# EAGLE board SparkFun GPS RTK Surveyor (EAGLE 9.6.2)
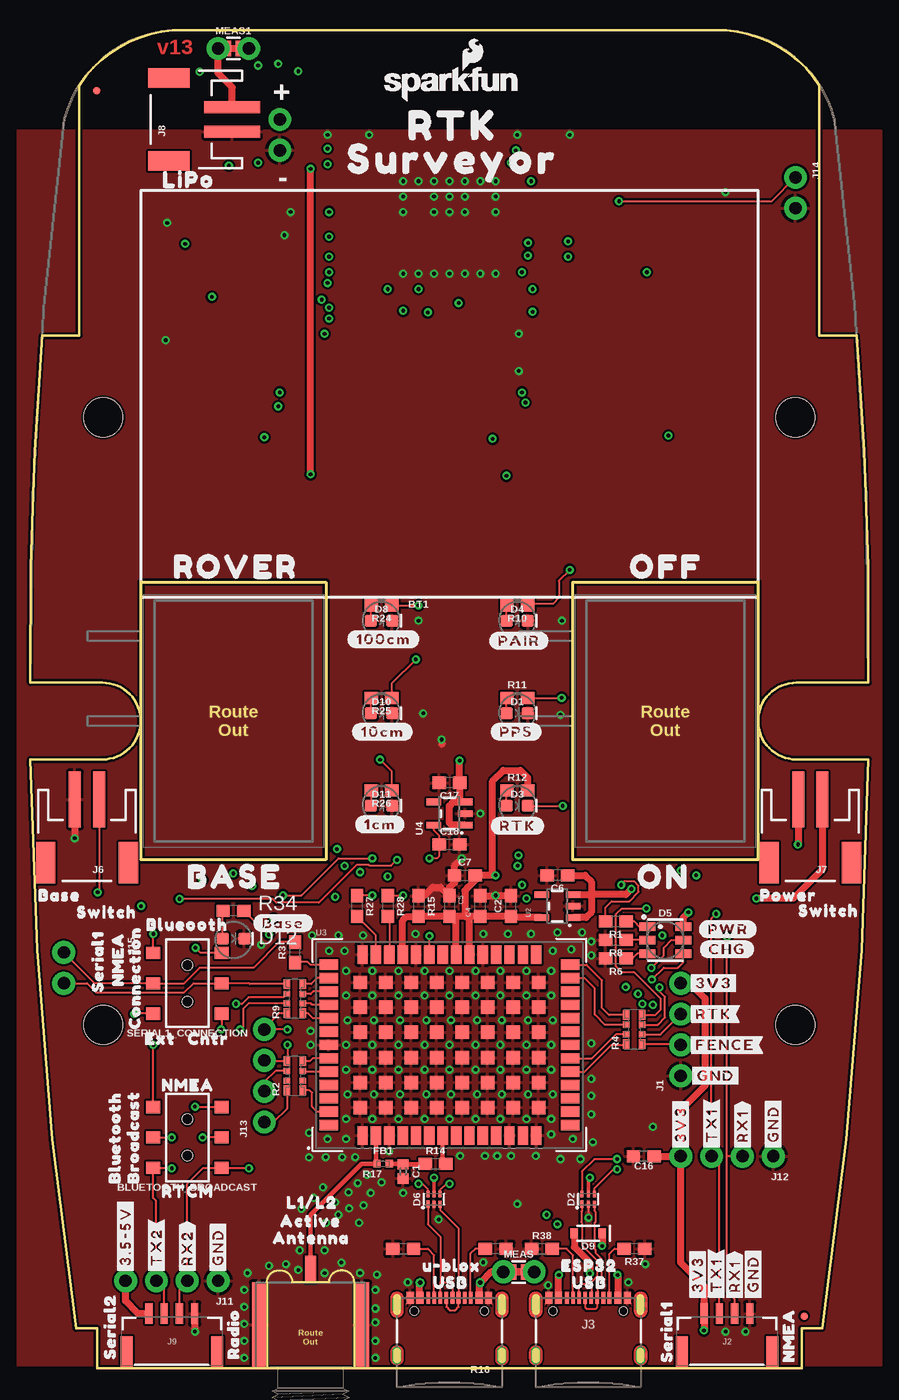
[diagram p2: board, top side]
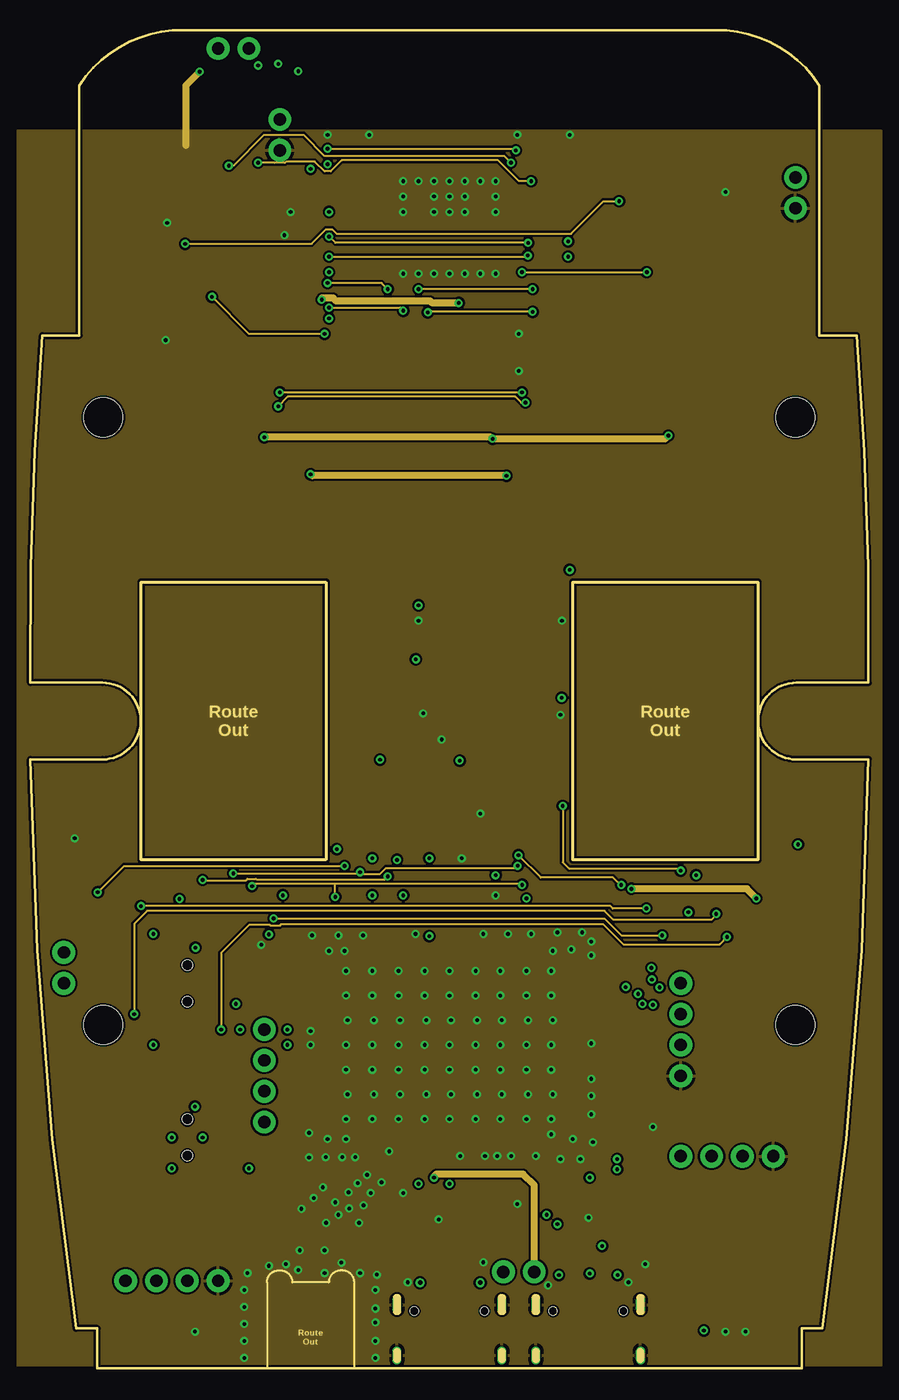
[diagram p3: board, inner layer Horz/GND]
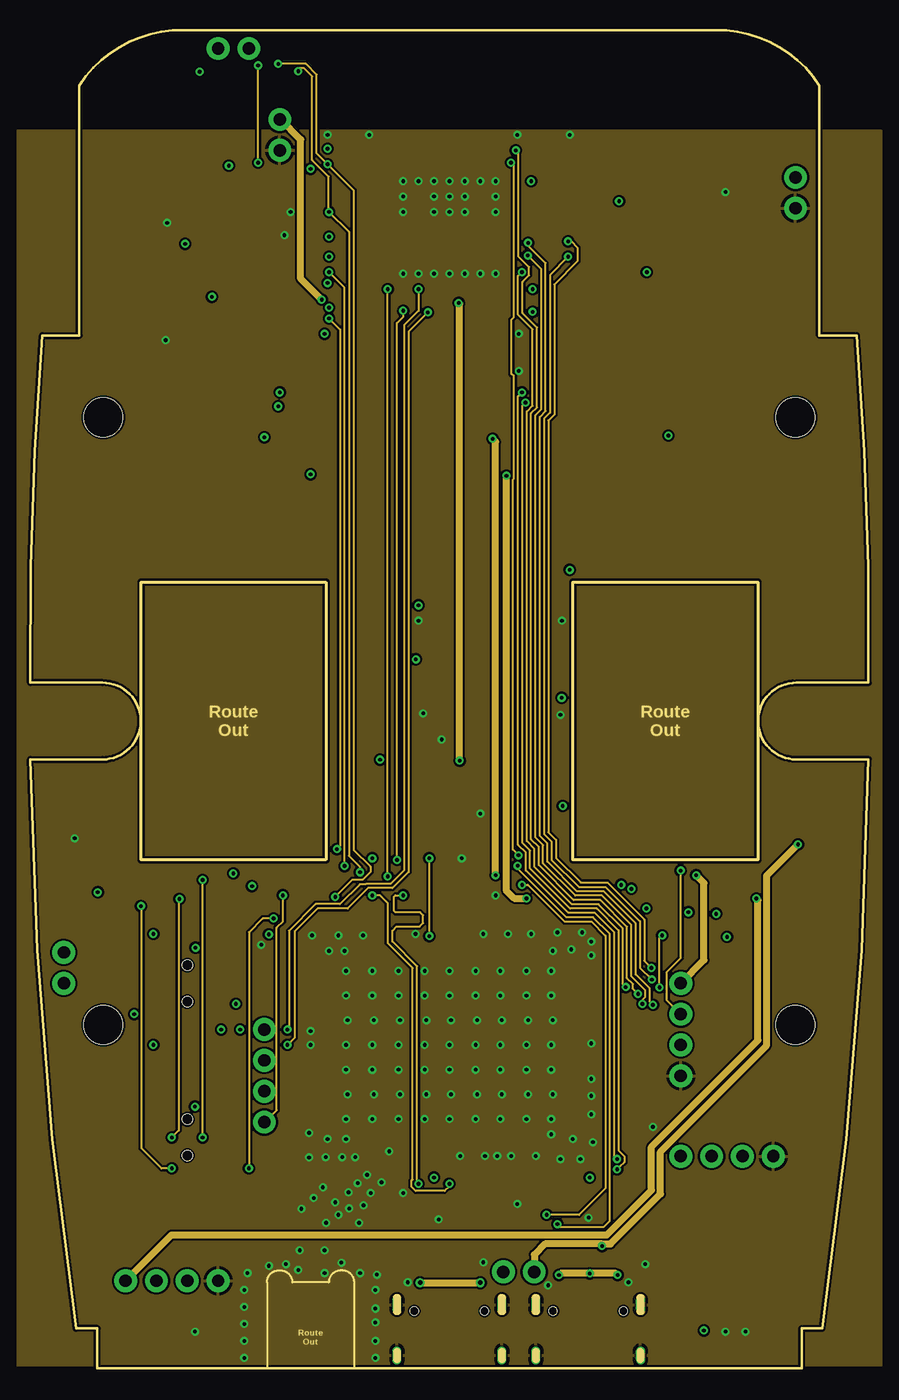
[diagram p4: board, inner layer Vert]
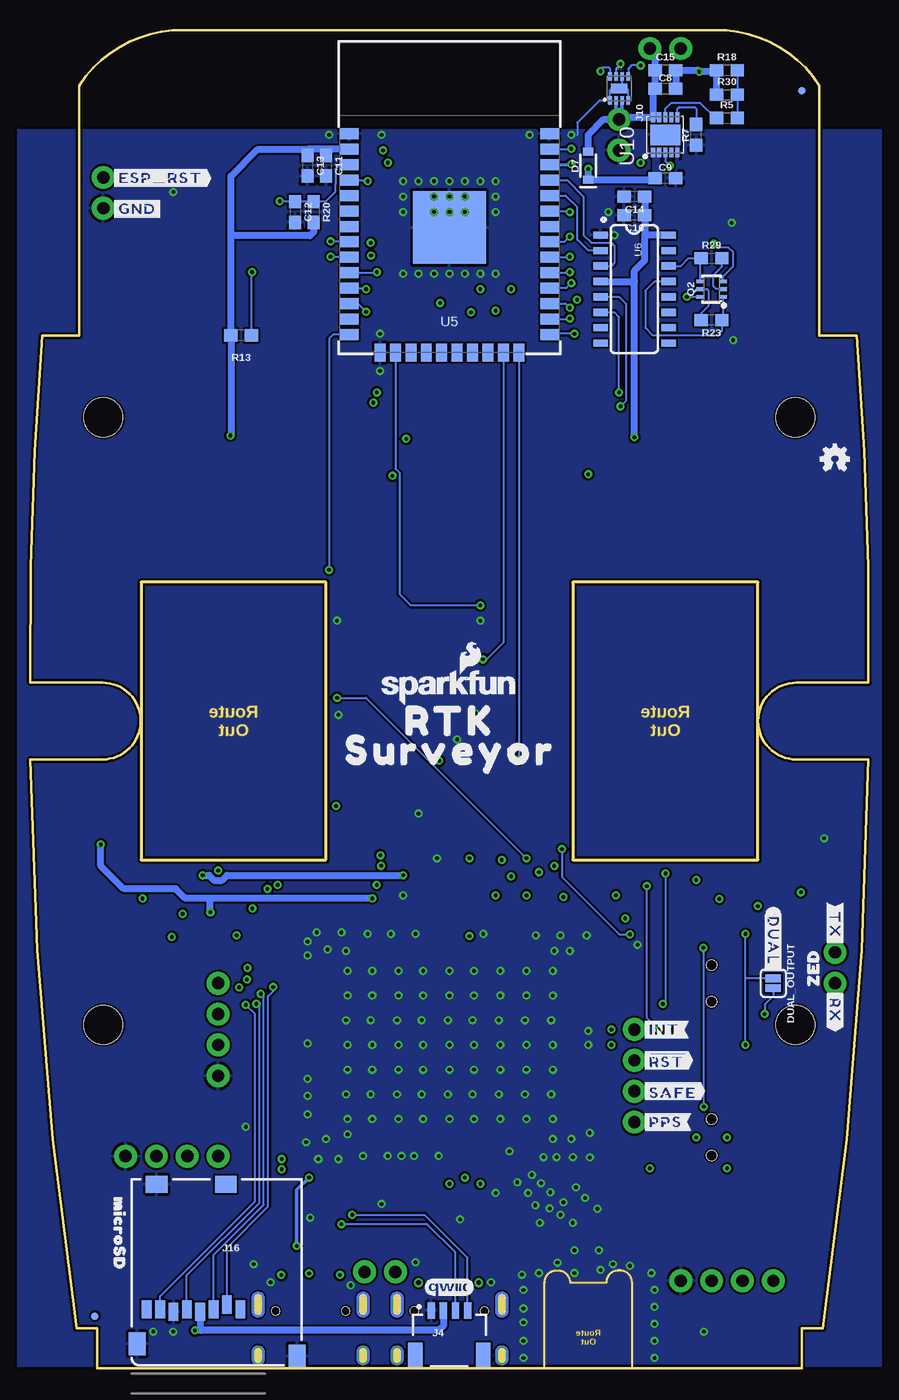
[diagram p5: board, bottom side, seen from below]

Size 69.02 x 110.14 mm. Coordinates in mm from the lower left corner, seen from the top.
Outline: 9.11,64.7 24.35,64.7 24.35,41.84 9.11,41.84 9.11,64.7
Outline: 44.67,64.7 59.91,64.7 59.91,41.84 44.67,41.84 44.67,64.7
Copper layers (1*2*15*16): Top 0.035559375mm / dielectric 0.47751875mm / Horz/GND 0.035559375mm / dielectric 0.47751875mm / Vert 0.035559375mm / dielectric 0.47751875mm / Bottom 0.035559375mm
Design rules "SparkFun-4-layer-TIGHT *": minimum track width 7mil, minimum drill 12mil, track to track 7mil, track to pad 7mil, pad to pad 7mil, via to via 7mil, smd to smd 7mil, copper to edge 7mil, drill to drill 7mil, minimum pad ring 7mil, minimum via ring 7mil, stop-mask expansion 4mil, vias tented up to drill 25mil, thermal gap 10mil
Net classes: 1 power: width 0.305 mm; 2 3.3V: width 0.559 mm; 3 RF: width 0.35 mm, clearance 0.203 mm

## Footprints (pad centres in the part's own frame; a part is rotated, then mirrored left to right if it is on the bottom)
SWITCH_DPDT_SMD_AYZ0202 = smd 1 x 1.15: 1 -2.5,2.825; 2 0,2.825; 3 2.5,2.825; 4 -2.5,-2.825; 5 0,-2.825; 6 2.5,-2.825 | hole 0.85: 1.5,0; -1.5,0
0402 = smd 0.85 x 0.9: 1 -0.58,0; 2 0.58,0
0603 = smd 1.1 x 1: 1 -0.85,0; 2 0.85,0
LED-0603 = smd 1 x 1: A -0.877,0; C 0.877,0
SOT886 = smd 0.61 x 0.25: 1 -0.405,0.5 | smd 0.56 x 0.25: 2 -0.43,0; 3 -0.43,-0.5; 4 0.43,-0.5; 5 0.43,0; 6 0.43,0.5
PLCC-6-LED = smd 1.3 x 0.7: AB 1.475,1.1; AG 1.475,-1.1; AR 1.475,0; CB -1.475,1.1; CG -1.475,-1.1; CR -1.475,0
SOD-323 = smd 0.63 x 0.83: A 1.15,0; C -1.15,0
SMT-JUMPER_2_NO_SILK = smd 0.635 x 1.27: 1 -0.406,0; 2 0.406,0
SMA-EDGE-SMD = smd 1.15 x 7: GND@0 -4.25,-3.5; GND@1 4.25,-3.5 | smd 0.9 x 2.2: SIG 0,-8.1
0402-TIGHT = smd 0.6 x 0.6: 1 -0.5,0; 2 0.5,0
1X04_NO_SILK = drill 1.016 pad 1.88: 1 0,0; 2 2.54,0; 3 5.08,0; 4 7.62,0
JST-4-SMD-1.25MM-LOCKING = smd 0.6 x 1.7: 1 -1.875,3.3; 2 -0.625,3.3; 3 0.625,3.3; 4 1.875,3.3 | smd 1 x 2.7: NC1 3.725,0.1; NC2 -3.725,0.1
USB-C-16P_4LAYER-PADS = smd 0.3 x 1: A5 -1.25,-0.34; A6 -0.25,-0.34; A7 0.25,-0.34; A8 1.25,-0.34; B5 1.75,-0.34; B6 0.75,-0.34; B7 -0.75,-0.34; B8 -1.75,-0.34 | smd 0.6 x 1: GND -3.225,-0.34; GND2 3.225,-0.34; VBUS1 -2.45,-0.34; VBUS2 2.45,-0.34 | drill 0.4 pad 0.6 long: SHLD1 -4.318,-0.915; SHLD2 4.318,-0.915; SHLD3 -4.318,-5.095; SHLD4 4.318,-5.095 | hole 0.65: -2.89,-1.445; 2.89,-1.445
JST04_1MM_RA = smd 0.6 x 1.35: 1 -1.5,0; 2 -0.5,0; 3 0.5,0; 4 1.5,0 | smd 1.2 x 2: NC1 2.8,-3.675; NC2 -2.8,-3.675
JST-2-SMD = smd 1 x 4.6: 1 -1,-3.7; 2 1,-3.7 | smd 1.6 x 3.4: NC1 -3.4,1.5; NC2 3.4,1.5
1X02_NO_SILK = drill 1.016 pad 1.88: 1 0,0; 2 2.54,0
MICRO-SD-SOCKET = smd 1.8 x 1.4: CD1 -2.05,0.4; CD2 -7.75,0.4 | smd 0.8 x 1.5: CS/DAT3 -7.84,10.3; DAT1 -1.24,10.7; DAT2 -8.94,10.7; DI/CMD -6.74,10.7; DO/DAT0 -2.34,10.7; GND -3.44,10.9; SCLK -4.54,10.7; VCC -5.64,10.9 | smd 1.4 x 1.9: GND1 -13.6,14.55; GND3 -0.45,13.55
FIDUCIAL-MICRO = smd 0.635 x 0.635: 1 0,0
COMBO-JUMPER_2_NC_TRACE = smd 0.635 x 1.27: 1 -0.508,0; 2 0.508,0 | drill 1.016 pad 1.88: 3 -1.27,0; 4 1.27,0
SC70-6 = smd 0.3 x 0.66: 1 -0.65,-0.92; 2 0,-0.92; 3 0.65,-0.92; 4 0.65,0.92; 5 0,0.92; 6 -0.65,0.92
1206_RA = smd 0.8 x 0.55: P1 -1.2,-0.62; P4 1.2,-0.62; P5 1.2,0.68; P8 -1.2,0.68 | smd 0.5 x 0.55: P2 -0.4,-0.62; P3 0.4,-0.62; P6 0.4,0.68; P7 -0.4,0.68
SOT23-5 = smd 0.55 x 1.2: 1 -0.95,-1.3; 2 0,-1.3; 3 0.95,-1.3; 4 0.95,1.3; 5 -0.95,1.3
ZED-F9P = smd 0.85 x 1.52: 1 -7.15,-7.45; 2 -6.05,-7.45; 3 -4.95,-7.45; 4 -3.85,-7.45; 5 -2.75,-7.45; 6 -1.65,-7.45; 7 -0.55,-7.45; 8 0.55,-7.45; 9 1.65,-7.45; 10 2.75,-7.45; 11 3.85,-7.45; 12 4.95,-7.45; 13 6.05,-7.45; 14 7.15,-7.45; 28 7.15,7.45; 29 6.05,7.45; 30 4.95,7.45; 31 3.85,7.45; 32 2.75,7.45; 33 1.65,7.45; 34 0.55,7.45; 35 -0.55,7.45; 36 -1.65,7.45; 37 -2.75,7.45; 38 -3.85,7.45; 39 -4.95,7.45; 40 -6.05,7.45; 41 -7.15,7.45 | smd 1.52 x 0.85: 15 9.95,-6.6; 16 9.95,-5.5; 17 9.95,-4.4; 18 9.95,-3.3; 19 9.95,-2.2; 20 9.95,-1.1; 21 9.95,0; 22 9.95,1.1; 23 9.95,2.2; 24 9.95,3.3; 25 9.95,4.4; 26 9.95,5.5; 27 9.95,6.6; 42 -9.95,6.6; 43 -9.95,5.5; 44 -9.95,4.4; 45 -9.95,3.3; 46 -9.95,2.2; 47 -9.95,1.1; 48 -9.95,0; 49 -9.95,-1.1; 50 -9.95,-2.2; 51 -9.95,-3.3; 52 -9.95,-4.4; 53 -9.95,-5.5; 54 -9.95,-6.6 | smd 1.1 x 1.1: 55 -1.05,-1.05; 56 -3.15,-1.05; 57 -5.25,-1.05; 58 -7.35,-1.05; 59 -1.05,-3.1; 60 -3.15,-3.1; 61 -5.25,-3.1; 62 -7.35,-3.1; 63 -1.05,-5.15; 64 -3.15,-5.15; 65 -5.25,-5.15; 66 -7.35,-5.15; 67 -1.05,5.15; 68 -3.15,5.15; 69 -5.25,5.15; 70 -7.35,5.15; 71 -1.05,3.1; 72 -3.15,3.1; 73 -5.25,3.1; 74 -7.35,3.1; 75 -1.05,1.05; 76 -3.15,1.05; 77 -5.25,1.05; 78 -7.35,1.05; 79 1.05,1.05; 80 3.15,1.05; 81 5.25,1.05; 82 7.35,1.05; 83 1.05,3.1; 84 3.15,3.1; 85 5.25,3.1; 86 7.35,3.1; 87 1.05,5.15; 88 3.15,5.15; 89 5.25,5.15; 90 7.35,5.15; 91 1.05,-5.15; 92 3.15,-5.15; 93 5.25,-5.15; 94 7.35,-5.15; 95 1.05,-3.1; 96 3.15,-3.1; 97 5.25,-3.1; 98 7.35,-3.1; 99 1.05,-1.05; 100 3.15,-1.05; 101 5.25,-1.05; 102 7.35,-1.05
ESP-WROOM-32-NARROW = smd 0.9 x 1.5: 1 6.43,8.238; 2 5.16,8.238; 3 3.89,8.238; 4 2.62,8.238; 5 1.35,8.238; 6 0.08,8.238; 7 -1.19,8.238; 8 -2.46,8.238; 9 -3.73,8.238; 10 -5,8.238; 11 -6.27,8.238; 12 -7.54,8.238; 13 -8.81,8.238; 14 -10.08,8.238; 25 -10.08,-8.238; 26 -8.81,-8.238; 27 -7.54,-8.238; 28 -6.27,-8.238; 29 -5,-8.238; 30 -3.73,-8.238; 31 -2.46,-8.238; 32 -1.19,-8.238; 33 0.08,-8.238; 34 1.35,-8.238; 35 2.62,-8.238; 36 3.89,-8.238; 37 5.16,-8.238; 38 6.43,-8.238 | smd 1.5 x 0.9: 15 -11.57,5.715; 16 -11.57,4.445; 17 -11.57,3.175; 18 -11.57,1.905; 19 -11.57,0.635; 20 -11.57,-0.635; 21 -11.57,-1.905; 22 -11.57,-3.175; 23 -11.57,-4.445; 24 -11.57,-5.715 | smd 6 x 6: GND -1.27,0
SO016 = smd 0.6 x 1.2: 1 -4.445,-2.8; 2 -3.175,-2.8; 3 -1.905,-2.8; 4 -0.635,-2.8; 5 0.635,-2.8; 6 1.905,-2.8; 7 3.175,-2.8; 8 4.445,-2.8; 9 4.445,2.8; 10 3.175,2.8; 11 1.905,2.8; 12 0.635,2.8; 13 -0.635,2.8; 14 -1.905,2.8; 15 -3.175,2.8; 16 -4.445,2.8
DFN-8 = smd 0.3 x 0.7: 1 -0.75,-0.99; 2 -0.25,-0.99; 3 0.25,-0.99; 4 0.75,-0.99; 5 0.75,0.99; 6 0.25,0.99; 7 -0.25,0.99; 8 -0.75,0.99 | smd 1.38 x 0.8: 9 0,0
DFN-10 = smd 0.8 x 0.35: 1 -1.45,1; 2 -1.45,0.5; 3 -1.45,0; 4 -1.45,-0.5; 5 -1.45,-1; 6 1.45,-1; 7 1.45,-0.5; 8 1.45,0; 9 1.45,0.5; 10 1.45,1 | smd 1.7 x 2.5: 11 0,0
1553DBK-ENCLOSURE = hole 3.2: -25.006,28.499; 25.006,28.499; 25.006,-28.499; -25.006,-28.499

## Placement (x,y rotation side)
BLUETOOTH_BROADCAST  [SWITCH_DPDT_SMD_AYZ0202]  12.92,18.98 90 top
BT1  LIPO-OUTLINE1100  [LIPO-1000]  59.91,63.43 90 top
C1  47pF  [0402]  30.7,16.19 270 top
C2  1.0uF  [0603]  39.59,38.03 90 top
C4  1.0uF  [0603]  37.05,38.03 90 top
C5  0.1uF  [0603]  34.51,38.03 270 top
C6  1.0uF  [0603]  43.4,40.57 180 top
C7  0.1uF  [0603]  35.78,40.57 0 top
C8  4.7uF  [0603]  16.73,105.34 0 bottom
C9  4.7uF  [0603]  16.73,97.98 0 bottom
C10  10uF  [0603]  19.27,94.93 180 bottom
C11  0.1uF  [0603]  44.67,99 270 bottom
C12  0.1uF  [0603]  47.21,95.19 270 bottom
C13  0.1uF  [0603]  46.19,99 270 bottom
C14  10uF  [0603]  19.27,96.45 180 bottom
C15  0.1uF  [0603]  16.73,106.87 0 bottom
C16  0.1uF  [0603]  50.51,17.44 180 top
C17  1.0uF  [0603]  34.51,48.19 180 top
C18  1.0uF  [0603]  34.51,43.11 0 top
D1  Yellow  [LED-0603]  40.1,53.91 0 top
D2  PRTR5V0U2F  [SOT886]  45.94,13.9 90 top
D3  WHITE  [LED-0603]  40.1,46.29 0 top
D4  BLUE  [LED-0603]  40.1,61.53 0 top
D5  RGB  [PLCC-6-LED]  52.29,35.24 0 top
D6  PRTR5V0U2F  [SOT886]  33.24,13.9 90 top
D7  3A/10V/280mV  [SOD-323]  23.08,99 90 bottom
D8  GREEN  [LED-0603]  28.92,61.53 0 top
D9  3A/10V/280mV  [SOD-323]  45.94,11.09 180 top
D10  GREEN  [LED-0603]  28.92,53.91 0 top
D11  GREEN  [LED-0603]  28.92,46.29 0 top
D12  RED  [LED-0603]  16.73,35.37 0 top
DUAL_OUTPUT  [SMT-JUMPER_2_NO_SILK]  7.84,31.68 270 bottom
E1  SMA  [SMA-EDGE-SMD]  23.08,0.05 180 top
FB1  2.66Ω  [0402-TIGHT]  29.05,16.83 0 top
FRAME1  FRAME-LETTERNO_PACKAGE  [DUMMY]  not placed on the board
FRAME2  FRAME-LEDGER  [CREATIVE_COMMONS]  not placed on the board
J1  [1X04_NO_SILK]  53.56,24.06 90 top
J2  [JST-4-SMD-1.25MM-LOCKING]  57.37,1.19 0 top
J3  USB Female Type C Connector  [USB-C-16P_4LAYER-PADS]  45.94,6.14 0 top
J4  Qwiic Right Angle  [JST04_1MM_RA]  34.51,4.74 0 bottom
J5  USB Female Type C Connector  [USB-C-16P_4LAYER-PADS]  34.51,6.14 0 top
J6  Start Base  [JST-2-SMD]  4.66,43.11 180 top
J7  Power Switch  [JST-2-SMD]  64.23,43.11 180 top
J8  [JST-2-SMD]  12.92,102.81 90 top
J9  [JST-4-SMD-1.25MM-LOCKING]  11.65,1.19 0 top
J10  [1X02_NO_SILK]  20.54,102.81 270 bottom
J11  [1X04_NO_SILK]  15.46,7.19 180 top
J12  [1X04_NO_SILK]  61.18,17.44 180 top
J13  [1X04_NO_SILK]  19.27,20.25 90 top
J14  [1X02_NO_SILK]  63.01,98.03 270 top
J15  [1X02_NO_SILK]  2.76,34.22 270 top
J16  microSD  [MICRO-SD-SOCKET]  60.67,15.54 180 bottom
JP21  FIDUCIALUFIDUCIAL  [FIDUCIAL-MICRO]  63.72,4.28 0 top
JP61  FIDUCIALUFIDUCIAL  [FIDUCIAL-MICRO]  5.48,105.16 0 top
JP71  FIDUCIALUFIDUCIAL  [FIDUCIAL-MICRO]  63.72,4.28 0 bottom
JP81  FIDUCIALUFIDUCIAL  [FIDUCIAL-MICRO]  5.48,105.16 0 bottom
LOGO1  OSHW-LOGOMINI  [OSHW-LOGO-MINI]  2.76,74.87 0 bottom
LOGO2  SFE_LOGO_NAME_FLAME.1_INCH  [SFE_LOGO_NAME_FLAME_.1]  34.51,56.07 0 bottom
LOGO3  SFE_LOGO_NAME_FLAME.1_INCH  [SFE_LOGO_NAME_FLAME_.1]  34.71,105.73 0 top
MEAS  [COMBO-JUMPER_2_NC_TRACE]  40.22,7.92 0 top
MEAS1  [COMBO-JUMPER_2_NC_TRACE]  16.73,108.65 0 top
Q2  MBT3904DW1T1  [SC70-6]  12.92,88.84 90 bottom
R1  4.7k  [0603]  48.23,36.76 180 top
R2  33  [1206_RA]  21.81,24.06 90 top
R3  33  [0603]  21.81,34.22 90 top
R4  33  [1206_RA]  49.75,27.87 90 top
R5  0  [0603]  11.65,102.93 0 bottom
R6  1k  [0603]  48.23,33.72 180 top
R7  1k  [0603]  14.19,101.53 90 bottom
R8  1k  [0603]  48.23,35.24 180 top
R9  33  [1206_RA]  21.81,30.41 90 top
R10  330  [0603]  40.1,62.8 180 top
R11  20  [0603]  40.1,55.18 0 top
R12  330  [0603]  40.1,47.56 0 top
R13  100k  [0603]  51.65,85.03 180 bottom
R14  10  [0603]  33.37,16.83 0 top
R15  100k  [0603]  31.97,38.03 270 top
R16  5.1k  [0603]  38.32,9.82 180 top
R17  5.1k  [0603]  30.7,9.82 0 top
R18  10k  [0603]  11.65,106.87 0 bottom
R20  10k  [0603]  45.69,95.19 270 bottom
R23  10k  [0603]  12.92,86.29 180 bottom
R24  20  [0603]  28.92,62.8 180 top
R25  20  [0603]  28.92,55.18 180 top
R26  20  [0603]  28.92,47.56 180 top
R27  27  [0603]  26.89,38.03 270 top
R28  27  [0603]  29.43,38.03 270 top
R29  10k  [0603]  12.92,91.38 0 bottom
R30  150k  [0603]  11.65,104.84 0 bottom
R34  330  [0603]  16.73,37.65 180 top
R37  5.1k  [0603]  49.75,9.82 180 top
R38  5.1k  [0603]  42.13,9.82 0 top
SERIAL1_CONNECTION  [SWITCH_DPDT_SMD_AYZ0202]  12.92,31.68 90 top
U2  3.3V  [SOT23-5]  43.4,38.03 90 top
U3  U-BLOX_ZED-F9P  [ZED-F9P]  34.51,26.6 0 top
U4  3.3V  [SOT23-5]  34.51,45.65 90 top
U5  ESP-WROOM-32NARROW  [ESP-WROOM-32-NARROW]  34.51,95.19 90 bottom
U6  CH340C  [SO016]  19.27,88.84 270 bottom
U7  MAX17048  [DFN-8]  20.54,105.34 0 bottom
U10  MCP73833  [DFN-10]  16.73,101.53 90 bottom
U$1  [#GND#0]  54.19,24.06 0 top
U$2  SPECIAL_INSTRUCTIONS-ORDERING  [ORDERING_INSTRUCTIONS]  not placed on the board
U$3  [ROCKER_SWITCH]  16.73,53.27 90 top
U$4  [#BASE#0]  18.38,36.64 0 top
U$5  [#3V3#0]  53.56,17.86 90 top
U$6  [ANTENNA0]  19.27,10.71 0 top
U$7  [RTK0]  34.51,53.27 0 bottom
U$8  [#CHG#0]  57.37,34.48 0 top
U$9  [_SURVEYOR3]  45.69,50.86 0 bottom
U$10  [#RTK#1]  54.07,29.14 0 top
U$11  [#PPS#0]  18.76,20.25 0 bottom
U$12  [#RTK#0]  37.94,44.64 0 top
U$13  [LIGHT_PIPE_3MM]  52.28,35.22 0 top
U$14  [#RX#2]  2.76,31.18 270 bottom
U$15  [LIGHT_PIPE_3MM]  16.73,35.25 0 top
U$16  [ZED0]  4.54,30.8 90 bottom
U$17  [##SAFE##5]  18.76,22.79 0 bottom
U$18  [ACTIVE0]  19.9,12.11 0 top
U$19  [L1#L21]  20.41,13.63 0 top
U$20  [#PAIR#0]  37.81,59.88 0 top
U$21  [LIGHT_PIPE_3MM]  28.91,46.37 0 top
U$22  [BASE2]  11.52,40.45 0 top
U$23  [#3#5#5V#0]  7.84,7.7 90 top
U$24  [#PPS#1]  37.94,52.39 0 top
U$25  [#PWR#2]  55.08,36.13 0 top
U$26  [1553DBK-ENCLOSURE]  34.51,53.27 90 top
U$27  [LIPO0]  13.05,97.85 0 top
U$28  [##RST##4]  18.76,25.33 0 bottom
U$29  [SERIAL10]  52.42,-0.18 90 top
U$30  [QWIIC_4MM]  34.51,6.65 0 bottom
U$31  [OFF1]  47.97,65.97 0 top
U$32  [#FENCE#3]  54.07,26.6 0 top
U$33  [#INT#0]  18.76,27.87 0 bottom
U$34  [ROCKER_SWITCH]  52.29,53.27 90 top
U$35  [U#BLOX0]  31.59,8.43 0 top
U$36  [USB1]  32.48,7.03 0 top
U$37  [#3V3#0]  54.07,31.68 0 top
U$38  [#GND#0]  15.46,7.7 90 top
U$39  [#RX2#2]  12.92,7.7 90 top
U$40  [#TX2#1]  10.38,7.7 90 top
U$41  [BLUETOOTH2]  6.95,14.54 90 top
U$42  [ON0]  48.61,40.45 0 top
U$43  [SERIAL20]  6.57,0.08 90 top
U$44  [ROVER3]  10.38,65.97 0 top
U$45  [#RX1#2]  58,5.51 90 top
U$46  [#TX1#1]  56.48,5.51 90 top
U$47  [#3V3#0]  54.96,5.51 90 top
U$48  [#GND#0]  59.53,5.51 90 top
U$49  [NMEA1]  62.45,-0.18 90 top
U$50  [RADIO0]  16.73,0.08 90 top
U$51  [BROADCAST3]  8.47,14.54 90 top
U$52  [NMEA1]  10.13,23.3 0 top
U$53  [RTCM0]  10.13,14.54 0 top
U$54  [BASE0]  -0.03,38.92 0 top
U$55  [SWITCH1]  3.14,37.53 0 top
U$56  [POWER0]  59.4,38.92 0 top
U$57  [SWITCH1]  62.58,37.65 0 top
U$58  [BLUEOOTH3]  8.86,36.51 0 top
U$59  [CNTR1]  12.28,27.11 0 top
U$60  [#ESP_RST#0]  62.45,97.98 0 bottom
U$61  [EXT0]  8.73,27.11 0 top
U$62  [NMEA2]  7.2,30.8 90 top
U$63  [SERIAL10]  5.55,30.29 90 top
U$64  [CONNECTION1]  8.6,27.24 90 top
U$65  [#TX1#1]  56.1,17.86 90 top
U$66  [USB1]  43.91,7.03 0 top
U$67  [ESP320]  43.02,8.43 0 top
U$68  [#RX1#2]  58.64,17.86 90 top
U$69  [LIGHT_PIPE_3MM]  40.11,46.37 0 top
U$71  [_SURVEYOR3]  23.51,99.53 0 top
U$72  [#TX#1]  2.76,38.29 270 bottom
U$73  [#DUAL#0]  7.84,37.91 270 bottom
U$74  [RTK0]  34.76,102.3 0 top
U$75  [LIGHT_PIPE_3MM]  40.11,53.97 0 top
U$76  [LIGHT_PIPE_3MM]  40.11,61.57 0 top
U$77  [LIGHT_PIPE_3MM]  28.91,61.57 0 top
U$78  [LIGHT_PIPE_3MM]  28.91,53.97 0 top
U$79  [#1CM#0]  26.76,44.77 0 top
U$80  [#10CM#1]  26.51,52.39 0 top
U$81  [#100CM#2]  26.13,60.01 0 top
U$82  [#GND#0]  61.18,17.86 90 top
U$83  [MICROSD0]  61.69,14.76 270 bottom
U$84  [#GND#1]  62.45,95.44 0 bottom

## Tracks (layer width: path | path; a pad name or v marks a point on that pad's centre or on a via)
3.3V  (via drill 0.3)
  Top 0.559: U2.5 39.69,37.08 C2.1 C4.1 36.16,37.18 | 36.16,37.18 35.78,37.18 | 35.78,37.18 35.14,37.18 | 35.14,37.18 C5.2 R15.2 30.99,37.18 30.66,36.85 U3.38 | 35.78,37.18 35.78,39.3 36.09,39.62 36.63,40.16 C7.2 38.07,40.57 | U3.34 35.06,37.1 35.14,37.18 | U3.33 36.16,37.18 | v38.32,40.57 38.07,40.57 | J1.4 54.32,31.68 55.55,30.45 55.55,23.25 53.56,21.25 J12.4 | R12.2 40.95,48.61 40.35,49.21 38.95,49.21 38.07,48.32 38.07,40.57 | J12.4 53.56,8.68 55.49,6.75 J2.1 55.49,3.12 v55.46,3.09 | C16.1 J12.4
  Horz/GND 0.559: v19.27,76.64 37.94,76.64 v38.07,76.52 52.29,76.52 v52.54,76.77
  Vert 0.559: v38.32,40.57 38.32,76.26 v38.07,76.52 | J1.4 55.46,33.59 55.46,39.94 v54.83,40.57
  Bottom 0.559: U5.2 44.67,100.34 | 44.67,100.34 46.19,100.34 | C13.1 46.19,100.34 | C11.1 44.67,100.34 | C14.1 C10.1 18.42,93.28 | 18.42,93.28 18.42,91.21 19.27,90.36 19.27,89.47 | U6.16 18.42,93.28 | v19.27,76.64 19.27,89.47 | U6.4 19.27,89.47 | v54.83,40.57 54.29,40.57 53.89,40.17 53.23,40.17 52.83,40.57 v38.32,40.57 | 46.19,100.34 50.3,100.34 52.5,98.14 52.5,93.28 | 52.5,93.28 R13.2 52.5,76.81 v52.54,76.77 | J4.2 35.01,3.48 35.4,3.09 54.96,3.09 | 54.96,3.09 v55.46,3.09 | J16.VCC 55.03,3.17 54.96,3.09 | 52.5,93.28 52.45,93.23 46,93.23 45.69,93.54 R20.2
5V  (via drill 0.3)
  Top 0.559: J9.1 8.89,4.49 7.84,5.54 J11.4 | v49.5,39.46 49.02,38.98 46.19,38.98 | U2.3 46.19,38.98 | C6.1 45.69,40.57 46.19,40.07 46.19,38.98 | 46.19,38.98 46.19,37.53 45.75,37.08 U2.1 | J7.1 65.23,41.07 62.83,38.67 v59.78,38.67
  Horz/GND 0.559: v49.5,39.46 59.02,39.46 59.02,39.43 v59.78,38.67
  Vert 0.559: v59.78,38.67 59.91,38.54 59.91,26.99 51.15,18.22 51.15,14.65 47.46,10.97 11.62,10.97 J11.4
ANT_VCC
  Top 0.351: FB1.2 30.64,16.83 C1.1 32.46,16.77 R14.1
BACKUP  (via drill 0.3)
  Top 0.178: U3.36 v32.86,35.57 | U4.5 33.21,44.29 33.66,43.84 C18.1 33.66,42.14 33.49,41.97 v32.86,41.97
  Vert 0.178: v32.86,35.57 v32.86,41.97
CC1
  Top 0.178: J5.A5 33.26,9.3 32.73,9.82 R17.2
CC2
  Top 0.178: J5.B5 36.26,9.45 36.64,9.82 R16.2
CC3
  Top 0.178: J3.B5 47.69,9.42 48.1,9.82 R37.2
CC4
  Top 0.178: J3.A5 44.69,9.3 44.16,9.82 R38.2
CHG_LED  (via drill 0.3)
  Top 0.178: R1.2 47.38,37.95 47.87,38.44 49.32,38.44 50.09,39.21 50.09,39.7 49.74,40.05 48.87,40.05 48.66,39.84 v48.66,39.79
  Horz/GND 0.178: v48.66,39.79 48.58,39.79 47.99,40.38 42.03,40.38 v40.2,42.22 | v39.58,99.25 39.03,99.79 24.23,99.79 22.49,101.53 19.27,101.53 16.73,99 v16.35,99
  Vert 0.178: v39.58,99.25 39.82,99.01 39.82,86.52 39.63,86.33 39.63,81.86 39.81,81.68 39.81,73.22 39.73,73.14 39.73,42.69 v40.2,42.22
  Bottom 0.178: U10.3 16.73,99.38 v16.35,99
CHG_THERM1
  Bottom 0.178: R18.2 R30.2 R5.2
D+  (via drill 0.3)
  Top 0.178: D6.4 33.74,14.66 34.26,15.17 v34.51,15.17 | R27.1 26.89,38.92 v28.16,38.92
  Vert 0.178: v34.51,15.17 34.51,14.97 34.12,14.58 31.72,14.58 31.37,14.93 31.37,15.42 31.49,15.54 31.49,32.93 29.43,34.99 29.43,38.29 28.79,38.92 v28.16,38.92
D+1  (via drill 0.3)
  Top 0.178: D2.4 46.44,14.79 48.02,16.37 v48.31,16.37
  Horz/GND 0.178: v40.77,79.49 40.43,79.49 39.95,79.97 21.2,79.97 v20.41,79.18
  Vert 0.178: v40.77,79.49 40.53,79.25 40.53,43.23 41.15,42.61 41.15,41.12 44.44,37.83 46.64,37.83 48.43,36.04 48.43,17.94 48.91,17.45 48.91,16.96 48.56,16.61 v48.31,16.37
  Bottom 0.178: U6.5 20.54,88.2 19.94,87.6 19.94,79.65 v20.41,79.18
D-  (via drill 0.3)
  Top 0.178: D6.6 32.74,14.72 32.28,15.17 v31.97,15.17 | v30.7,38.92 30.66,38.88 R28.1
  Vert 0.178: v31.97,15.17 31.84,15.3 31.84,33.08 29.81,35.11 29.81,36 30.15,36.35 32.06,36.35 32.35,36.64 32.35,37.27 32.1,37.53 30.06,37.53 29.94,37.65 29.94,38.8 30.06,38.92 v30.7,38.92
D-1  (via drill 0.3)
  Top 0.178: v48.31,17.21 46.45,17.21 45.43,16.19 D2.6
  Horz/GND 0.178: v40.48,80.33 v20.54,80.33
  Vert 0.178: v40.48,80.33 40.17,80.02 40.17,43.09 40.8,42.46 40.8,40.97 44.29,37.48 46.49,37.48 48.07,35.89 48.07,17.45 v48.31,17.21
  Bottom 0.178: U6.6 20.92,86.93 20.54,86.55 v20.54,80.33
ESP32_!DTR
  Bottom 0.178: Q2.1 12,86.37 R23.1 12.07,85.37 12.41,85.03 17.75,85.03 18.38,85.66 18.38,88.71 17.62,89.47 U6.13
ESP32_!RTS
  Bottom 0.178: Q2.4 13.84,91.31 R29.1 14.82,91.38 15.46,90.74 U6.14
ESP32_EN  (via drill 0.3)
  Top 0.178: J14.1 61.05,96.07 v48.48,96.07
  Horz/GND 0.178: v12.75,92.56 23.16,92.56 24.36,93.75 24.85,93.75 25.22,93.39 44.52,93.39 47.21,96.07 v48.48,96.07
  Bottom 0.178: Q2.3 12,89.88 11.14,90.74 11.14,91.88 11.52,92.26 12.45,92.26 v12.75,92.56 | U5.3 43.57,99.07 43.9,98.75 43.9,97.48 43.91,97.48 43.91,96.84 44.71,96.03 R20.1 C12.1 48.44,96.03 v48.48,96.07
ESP32_RXI
  Bottom 0.178: U5.34 24.94,96.53 23.97,95.57 23.97,92.9 23.08,92.01 U6.2
ESP32_TXO
  Bottom 0.178: U6.3 21.17,90.74 20.92,90.99 20.92,92.39 21.17,92.64 22.83,92.64 23.46,93.28 23.46,96.45 24.81,97.81 U5.35
ESP_0/BOOT  (via drill 0.3)
  Horz/GND 0.178: v14.95,88.2 17.96,85.19 24.18,85.19 v24.22,85.15
  Bottom 0.178: Q2.6 14.94,88.19 v14.95,88.2 | v24.22,85.15 26.22,85.15 U5.25
ESP_2/LED_1CM  (via drill 0.3)
  Top 0.178: R26.1 29.77,49.12 v28.79,50.1
  Bottom 0.178: U5.24 v28.79,50.1
ESP_4/LED_BASE_STAT  (via drill 0.3)
  Top 0.178: R34.1 17.62,37.65 19.56,35.71 v19.65,35.71
  Vert 0.178: v24.6,86.42 25.52,85.51 25.52,43.01 v25.24,42.73
  Bottom 0.178: U5.26 24.65,86.38 v24.6,86.42 | v25.24,42.73 25.24,40.45 20.5,35.71 v19.65,35.71
ESP_5/SWITCH_BASE_SELECT  (via drill 0.3)
  Top 0.178: J6.1 5.66,39.29 v5.55,39.18
  Horz/GND 0.178: v5.55,39.18 7.71,41.34 v25.87,41.34
  Vert 0.178: v25.87,41.34 25.87,88.96 v24.6,90.23
  Bottom 0.178: U5.29 24.65,90.19 v24.6,90.23
ESP_12/LED_BLUETOOTH  (via drill 0.3)
  Top 0.178: R10.1 40.95,62.93 43.02,62.93 43.53,63.43 43.53,64.83 v44.42,65.72
  Bottom 0.178: U5.14 44.08,85.1 44.42,84.77 v44.42,65.72
ESP_13/LED_100CM  (via drill 0.3)
  Top 0.178: R24.1 v31.97,62.8
  Bottom 0.178: v31.97,62.8 37.68,62.8 38.61,63.73 38.61,73.72 38.95,74.06 U5.16
ESP_15/LED_10CM  (via drill 0.3)
  Top 0.178: R25.1 29.77,56.39 v31.74,58.35
  Bottom 0.178: U5.23 30.06,59.75 31.46,58.35 v31.74,58.35
ESP_16/BT_RXI  (via drill 0.3)
  Top 0.178: v12.28,38.63 19.95,38.63 20.25,38.33 23.76,38.33 26.89,41.45 27.84,41.45 27.91,41.37 29.72,41.37 v30.19,41.84 | BLUETOOTH_BROADCAST.2 v11.65,18.98
  Horz/GND 0.178: v24.6,87.31 30.45,87.31 v30.7,87.06
  Vert 0.178: v11.65,18.98 12.23,19.56 12.23,38.57 v12.28,38.63 | v30.19,41.84 30.19,86.04 30.7,86.55 v30.7,87.06
  Bottom 0.178: U5.27 24.94,87.64 v24.6,87.31
ESP_17/BT_TXO  (via drill 0.3)
  Top 0.178: BLUETOOTH_BROADCAST.5 v14.19,18.98
  Horz/GND 0.178: v29.43,40.47 29.19,40.23 18.64,40.23 18.59,40.28 17.88,40.28 17.72,40.13 14.26,40.13 v14.19,40.19 | v29.43,88.84 28.92,89.34 v24.48,89.34
  Vert 0.178: v14.19,18.98 v14.19,40.19 | v29.43,40.47 v29.43,88.84
  Bottom 0.178: v24.48,89.34 24.9,88.91 U5.28
ESP_18/SD_SCK  (via drill 0.3)
  Horz/GND 0.178: v40.96,91.61 40.86,91.5 v24.6,91.5
  Vert 0.178: v50.41,29.98 50.41,30.32 50.64,30.55 50.64,31.11 49.5,32.25 49.5,36.48 47.08,38.9 44.88,38.9 42.22,41.56 42.22,43.05 41.6,43.68 41.6,78.46 42.08,78.95 42.08,90.49 v40.96,91.61
  Bottom 0.178: U5.30 24.65,91.45 v24.6,91.5 | J16.SCLK 56.13,7.62 50.16,13.6 50.16,29.75 50.38,29.98 v50.41,29.98
ESP_19/SD_CIPO  (via drill 0.3)
  Horz/GND 0.178: v40.99,92.64 25.12,92.64 v24.6,93.16
  Vert 0.178: v51.27,29.91 51,30.18 51,31.24 49.85,32.4 49.85,36.63 47.23,39.25 45.03,39.25 42.57,41.71 42.57,43.2 41.95,43.82 41.95,78.32 42.43,78.8 42.43,90.98 40.99,92.43 v40.99,92.64
  Bottom 0.178: v24.6,93.16 25.04,92.72 U5.31 | J16.DO/DAT0 58.33,5.93 50.51,13.75 50.51,29.14 v51.27,29.91
ESP_21/SDA  (via drill 0.3)
  Top 0.178: R9.P6 20.85,30.53 17.97,30.53 17.42,29.98 v16.93,29.98
  Horz/GND 0.178: 27.14,40.7 16.73,40.7 v16.71,40.72 | v40.12,41.36 39.93,41.17 29.28,41.17 28.81,40.7 27.14,40.7 | v27.14,40.83 27.14,40.7
  Vert 0.178: v27.14,40.83 27.14,41.25 26.23,42.17 26.23,93.56 v24.6,95.19 24.57,95.22 24.57,98.1 23.21,99.46 23.21,106.36 22.55,107.02 22.19,107.02 22.06,106.89 v22.06,106.78 | v43.4,11.86 43.65,11.6 47.21,11.6 47.72,12.11 47.72,35.75 46.34,37.12 44.14,37.12 40.12,41.14 v40.12,41.36
  Bottom 0.178: v16.93,29.98 16.73,30.19 16.73,40.7 v16.71,40.72 | U5.33 24.68,95.26 v24.6,95.19 | J4.3 34.01,9.52 36.35,11.86 v43.4,11.86 | v22.06,106.78 22.06,106.91 21.85,107.12 21.43,107.12 21.29,106.98 U7.8
ESP_22/SCL  (via drill 0.3)
  Top 0.178: R9.P7 17.95,30.01 17.53,29.59 17.53,28.13 v17.28,27.87
  Horz/GND 0.178: v40.5,39.79 40.41,39.88 25.11,39.88 | 25.11,39.88 18.44,39.88 v18.25,39.69 | v25.11,38.8 25.11,39.88
  Vert 0.178: v42.51,12.62 45.18,12.62 47.36,14.8 47.36,35.6 46.2,36.76 44,36.76 40.98,39.79 v40.5,39.79 | v25.11,38.8 26.51,40.19 27.35,40.19 27.99,40.84 27.99,41.28 26.64,42.64 26.64,96.96 v24.48,99.12 23.59,100.01 23.59,106.49 22.7,107.38 v20.41,107.38
  Bottom 0.178: v17.28,27.87 18.25,28.85 v18.25,39.69 | J4.4 33.01,9.09 36.54,12.62 v42.51,12.62 | v20.41,107.38 20.79,107 U7.7
  Bottom 0.254: U5.36 24.52,99.07 v24.48,99.12
ESP_23/SD_COPI  (via drill 0.3)
  Horz/GND 0.178: v24.48,100.39 39.84,100.39 v39.97,100.26
  Vert 0.178: v50.04,30.8 49.62,31.22 49.62,31.62 49.14,32.1 49.14,36.34 46.93,38.54 44.73,38.54 41.86,41.41 41.86,42.91 41.24,43.53 41.24,78.61 41.72,79.09 41.72,85.68 40.53,86.87 40.53,89.44 41.08,89.98 41.08,90.65 40.17,91.55 40.17,100.06 v39.97,100.26
  Bottom 0.178: J16.DI/CMD 53.93,9.32 49.8,13.45 49.8,30.56 v50.04,30.8 | U5.37 24.52,100.34 v24.48,100.39
ESP_25/SD_!CS!  (via drill 0.3)
  Horz/GND 0.178: v40.48,90.23 v50.77,90.23
  Vert 0.178: v49.03,31.37 48.78,31.61 48.78,36.19 46.79,38.19 44.59,38.19 41.51,41.27 41.51,42.76 40.88,43.38 40.88,78.76 41.37,79.24 41.37,85.53 40.17,86.73 40.17,89.93 v40.48,90.23
  Bottom 0.178: U5.10 40.53,90.19 v40.48,90.23 | R13.1 50.8,90.19 v50.77,90.23 | v49.03,31.37 49.03,31.03 49.44,30.61 49.44,13.3 52.83,9.92 J16.CS/DAT3
ESP_26/ZED_TX_READY  (via drill 0.3)
  Top 0.178: R9.P8 20.48,29.21 19.27,28 J13.4 v21.17,27.87
  Horz/GND 0.178: v41.37,88.84 v31.97,88.84
  Vert 0.178: v31.97,88.84 31.97,87.06 30.79,85.88 30.79,40.99 29.68,39.88 27.66,39.88 27.62,39.84 27.13,39.84 25.49,38.2 23.5,38.2 21.3,36 21.3,28 v21.17,27.87
  Bottom 0.178: U5.11 41.45,88.91 v41.37,88.84
ESP_27/ZED_!RESET!  (via drill 0.3)
  Top 0.178: J13.3 19.34,25.26 R2.P5 21.17,25.31 v21.17,26.6
  Horz/GND 0.178: v41.37,86.97 32.77,86.97 v32.73,86.93
  Vert 0.178: v21.17,26.6 21.77,27.2 21.77,35.97 23.65,37.84 26.13,37.84 27.8,39.52 29.82,39.52 31.14,40.84 31.14,85.34 v32.73,86.93
  Bottom 0.178: U5.12 42.04,87.64 v41.37,86.97
ESP_32/PWR_LVL_RED  (via drill 0.3)
  Top 0.178: v51.15,32.95 52.16,33.97 52.16,34.61 52.8,35.24 D5.AR
  Vert 0.178: v44.29,92.77 44.54,92.77 45.05,92.26 45.05,91.12 43.15,89.22 43.15,78.5 42.66,78.02 42.66,44.12 43.29,43.5 43.29,42 45.32,39.96 47.52,39.96 50.56,36.92 50.56,33.54 v51.15,32.95
  Bottom 0.178: U5.8 44.24,92.72 v44.29,92.77
ESP_33/PWR_LVL_GRN  (via drill 0.3)
  Top 0.178: v51.18,31.98 52.16,32.95 53.31,32.95 53.76,33.41 D5.AG
  Vert 0.178: v44.29,91.5 42.79,90 42.79,78.65 42.31,78.17 42.31,43.97 42.93,43.35 42.93,41.86 45.18,39.61 47.37,39.61 50.21,36.78 50.21,32.96 v51.18,31.98
  Bottom 0.178: U5.9 44.24,91.45 v44.29,91.5
ESP_36/BATT_ALRT  (via drill 0.3)
  Horz/GND 0.178: v41.24,97.72 40.22,97.72 38.51,99.44 25.64,99.44 24.72,98.53 24.23,98.53 23.42,99.34 21.07,99.34 20.97,99.24 20.11,99.24 20.1,99.25 v18.76,99.25
  Vert 0.178: v18.76,99.25 v18.76,107.25
  Bottom 0.178: U5.4 41.32,97.81 v41.24,97.72 | v18.76,107.25 19.52,107.25 19.79,106.98 U7.5
ESP_D1+
  Top 0.178: D2.3 46.44,12.97 46.57,12.84 46.57,12.06 46.49,11.98 46.49,9.81 46.57,9.72 46.57,9.46 47.02,9.01 47.02,7.4 46.69,7.07 J3.B6 46.69,5 46.57,4.89 45.81,4.89 45.69,5.01 J3.A6
ESP_D1-
  Top 0.178: 46.19,6.92 46.19,7.07 46.66,7.55 46.66,8.87 45.44,10.09 45.44,11.94 45.37,12.01 45.37,12.87 45.44,12.94 D2.1 | 46.19,6.92 J3.A7 | J3.B7 45.19,6.68 45.43,6.92 46.19,6.92
EXTERNAL_SERIAL1_RXI  (via drill 0.3)
  Top 0.178: 57.37,17.44 57.37,6.28 57.99,5.66 J2.3 | v15.71,27.87 15.74,27.91 SERIAL1_CONNECTION.4 | J12.2 57.37,17.44 | 57.37,17.44 v57.37,35.49
  Horz/GND 0.178: v15.71,27.87 15.71,34.19 18,36.47 19.73,36.47 19.78,36.42 20.53,36.42 20.62,36.51 47.21,36.51 48.82,34.9 56.77,34.9 v57.37,35.49
EXTERNAL_SERIAL1_TXO  (via drill 0.3)
  Top 0.178: v8.55,29.14 8.59,29.18 SERIAL1_CONNECTION.1 | v56.48,37.4 56.1,37.02 J12.3 56.74,16.8 J2.2
  Horz/GND 0.178: v56.48,37.4 56.48,37.29 56.09,36.9 48.03,36.9 47.28,37.65 9.62,37.65 8.55,36.59 v8.55,29.14
  Bottom 0.178: DUAL_OUTPUT.2 7.84,30.64 8.55,29.93 v8.55,29.14
FENCE_LV
  Top 0.178: U3.19 45.64,24.4 47.84,26.6 49,26.6 R4.P8
GND  (via drill 0.3)
  Top 0.178: D2.2 45.94,12.41 v45.97,12.38
  Top 0.559: C4.2 38.28,38.88 | 38.28,38.88 v38.32,38.92 | C2.2 38.28,38.88 | v35.53,41.97 34.93,41.38 C7.1 34.93,39.98 34.51,39.56 C5.1 34.48,38.88 33.78,39.58 33.13,39.58 32.43,38.88 R15.1 | 33.91,51.4 33.87,51.37 | J9.4 13.52,3.03 v13.55,3 | J6.2 3.66,43.64 v3.65,43.62
  Horz/GND 0.559: v13.94,106.74 12.79,105.6 12.79,100.65
  Bottom 0.178: U7.4 19.79,105.23 19.9,105.34 20.29,105.34 | 20.29,105.34 U7.9 21.17,105.34 21.29,105.23 U7.1 22.16,104.35 23.97,102.55 23.97,101.53 | U7.6 20.29,105.35 20.29,105.34
  Bottom 0.559: C8.2 C15.2 14.06,106.87 v13.94,106.74 12.63,106.74 R18.1 R30.1
  other vias: 42.64,6.81 57.24,3 30.7,14.41 33.62,12.24 37.3,8.71 31.08,7.06 11.27,94.3 11.14,84.64 21.43,95.19 20.92,93.28 28.29,28.64 30.45,28.64 32.6,28.64 34.64,28.64 36.8,28.64 38.83,28.64 40.99,28.64 43.02,28.64 26.13,28.64 28.16,30.67 30.32,30.67 32.48,30.67 34.51,30.67 36.67,30.67 38.7,30.67 40.86,30.67 42.89,30.67 26,30.67 28.16,32.7 30.32,32.7 32.48,32.7 34.51,32.7 36.67,32.7 38.7,32.7 40.86,32.7 42.89,32.7 26,32.7 28.29,22.54 30.45,22.54 32.6,22.54 34.64,22.54 36.8,22.54 38.83,22.54 40.99,22.54 43.02,22.54 26.13,22.54 28.16,24.57 30.32,24.57 32.48,24.57 34.51,24.57 36.67,24.57 38.7,24.57 40.86,24.57 42.89,24.57 26,24.57 28.16,26.6 30.32,26.6 32.48,26.6 34.51,26.6 36.67,26.6 38.7,26.6 40.86,26.6 42.89,26.6 26,26.6 28.16,20.51 30.32,20.51 32.48,20.51 34.51,20.51 36.67,20.51 38.7,20.51 40.86,20.51 42.89,20.51 26,20.51 25.68,17.36 38.45,17.46 35.4,17.46 37.43,17.46 39.59,17.46 41.62,17.46 24.33,17.36 23.21,35.62 25.37,35.62 27.4,35.62 31.72,35.75 37.3,35.75 39.34,35.75 41.24,35.75 43.4,35.88 45.43,35.88 46.19,33.97 46.19,26.73 46.19,23.81 46.19,22.41 46.19,20.89 46.32,18.6 46.19,35.11 42.89,19.24 45.3,17.21 43.65,17.21 26.75,17.36 27.72,15.92 26.96,15.23 26.2,14.47 25.11,13.65 24.1,14.89 23.33,14 24.35,11.96 22.06,8.08 21.05,8.55 25.62,8.68 19.65,8.43 17.87,7.82 24.22,7.82 17.62,6.43 17.62,5.03 17.62,3.63 17.62,0.84 17.62,2.24 25.37,12.62 26.25,13.13 22.95,17.33 22.95,19.37 24.48,18.86 23.08,26.6 23.08,27.75 22.32,13.11 27.44,13.4 28.03,14.41 28.92,15.3 27.07,11.96 27.14,7.82 28.54,7.7 28.41,6.43 28.41,4.9 28.41,3.76 28.41,2.24 28.41,0.84 29.56,17.84 26,18.86 25.87,34.35 24.6,34.35 43.02,34.35 44.54,34.48 44.67,18.86 33.87,51.75 22.19,9.7 24.22,9.7 57.24,96.84 43.65,53.78 32.35,53.91 31.97,61.53 43.78,61.53 30.7,95.19 30.7,96.45 38.32,96.45 38.32,95.19 37.05,90.1 35.78,90.1 34.51,90.1 33.24,90.1 31.97,90.1 30.7,90.1 30.7,97.72 31.97,97.72 33.24,97.72 34.51,97.72 35.78,97.72 37.05,97.72 38.32,97.72 38.32,90.1 33.24,96.45 33.24,95.19 34.51,95.19 34.51,96.45 35.78,96.45 35.78,95.19 58.89,3 49.24,7.06 24.48,101.53 44.42,101.53 40.1,101.53 27.91,101.53 40.22,85.15 40.22,82.1 37.05,45.65 19.02,34.86 51.27,19.86 50.64,8.55 40.1,13.51
  pour Top (isolate 0.152, rank 4): -1.05,101.91 70.07,101.91 70.07,0.2 -1.05,0.2
  pour Bottom (isolate 0.152, rank 4): -1.05,101.91 70.07,101.91 70.07,0.2 -1.05,0.2
  pour Horz/GND (isolate 0.152, rank 4): -1.05,101.91 70.07,101.91 70.07,0.17 -1.05,0.17
  pour Vert (isolate 0.152, rank 4): -1.05,101.91 70.07,101.91 70.07,0.17 -1.05,0.17
GPS_ANT1
  Top 0.35: 23.08,12.6 23.08,12.62 27.28,16.83 FB1.1 28.46,16.91 28.46,17.98
  Top 0.351: U3.2 28.46,17.98 | 23.08,12.6 E1.SIG
LIPO_RAW
  Top 0.559: J8.2 16.62,105.45 15.46,106.62 MEAS1.3 MEAS1.1
N$1
  Top 0.178: D3.A 39.22,47.53 R12.1
N$2
  Top 0.178: D1.A 39.22,55.15 R11.1
N$3
  Top 0.178: D4.A 39.22,62.77 R10.2
N$4  (via drill 0.38)
  Top 0.559: J5.VBUS1 32.06,6.99 v32.1,7.03 | J5.VBUS2 36.96,6.94 v37.05,7.03 37.94,7.92 MEAS.3 MEAS.1
  Vert 0.559: v32.1,7.03 v37.05,7.03
N$5
  Bottom 0.178: U10.8 16.73,103.69 16.25,104.18 13.87,104.18 12.63,102.93 R5.1
N$10
  Top 0.178: D5.CG 50.01,34.14 49.58,33.72 R6.1
N$11
  Top 0.178: U3.40 28.46,35.61 R27.2
N$12
  Top 0.178: R28.2 29.56,37.05 U3.39
N$13
  Top 0.351: U3.7 33.96,17.08 R14.2
N$14
  Top 0.178: D5.CR R8.1
N$16
  Top 0.178: U3.49 23.25,25.5 23.01,25.26 R2.P4
N$17
  Top 0.178: D5.CB 50.17,36.34 49.75,36.76 R1.1
N$18
  Top 0.178: U3.50 22.49,24.4 R2.P3
N$22
  Top 0.178: U3.46 23.29,28.8 22.88,29.21 R9.P1
N$24
  Bottom 0.178: Q2.5 13.3,88.84 13.17,88.71 13.17,87.44 13.77,86.84 R23.2
N$25
  Bottom 0.178: Q2.2 12.54,88.84 12.79,89.09 12.79,89.98 12.07,90.7 R29.2
N$26
  Top 0.178: D8.A 28.04,62.77 R24.2
N$27
  Top 0.178: D10.A 28.04,55.15 R25.2
N$29
  Top 0.178: R26.2 28.07,46.32 D11.A
N$30
  Top 0.178: D12.A 15.85,37.63 R34.2
N$32  (via drill 0.3)
  Top 0.559: J3.VBUS1 43.49,7.63 v43.53,7.67 | v48.35,7.67 48.39,7.63 J3.VBUS2 | D9.A 44.79,9.97 46.07,8.69 v46.07,7.79
  Vert 0.559: v43.53,7.67 43.65,7.79 v46.07,7.79 48.23,7.79 v48.35,7.67
NMEA-RX  (via drill 0.3)
  Top 0.178: SERIAL1_CONNECTION.6 14.01,34.18 v13.59,34.61 | v13.55,21.52 15.7,21.52 BLUETOOTH_BROADCAST.6
  Bottom 0.178: v13.59,34.61 13.59,33.49 13.61,33.47 13.61,21.58 v13.55,21.52
NMEA-TX  (via drill 0.3)
  Top 0.178: BLUETOOTH_BROADCAST.3 10.09,26.57 v10.13,26.6 | SERIAL1_CONNECTION.3 10.13,34.22 v10.13,35.75
  Bottom 0.178: v10.13,26.6 10.13,32.07 | 10.13,32.07 v10.13,35.75 | DUAL_OUTPUT.1 10.1,32.09 10.13,32.07
PPS
  Top 0.178: U3.53 23.63,21.1 23.21,21.52 23.21,22.67 23.01,22.86 R2.P1
PROG1
  Bottom 0.178: U10.6 15.73,103.68 15.59,103.82 14.32,103.82 14.19,103.69 R7.2
RTK_LV
  Top 0.178: U3.20 46.24,25.5 48.21,27.47 R4.P7
RX2_LV
  Top 0.178: U3.26 45.65,32.1 46.49,31.26 46.49,29.11 47.32,28.27 R4.P6
RXLV
  Top 0.178: U3.43 23.63,32.1 23.14,31.61 R9.P4
SCL_LV
  Top 0.178: U3.45 23.21,29.9 23.1,30.01 R9.P2
SDA_LV
  Top 0.178: U3.44 23.29,31 23.08,30.8 22.45,30.8 R9.P3
TX2_LV
  Top 0.178: U3.27 45.81,33.2 47.08,31.93 47.08,29.65 47.66,29.07 R4.P5
TXLV
  Top 0.178: U3.42 23.08,33.2 22.83,33.46 21.9,33.46 R3.1
UNP_D+
  Top 0.178: J5.A6 34.26,5.03 34.51,4.78 35.02,4.78 35.27,5.03 35.27,5.79 | 35.27,5.79 J5.B6 | D6.3 33.74,13.02 35.27,11.49 35.27,5.79
UNP_D-
  Top 0.178: 33.76,7.06 34.51,7.06 34.76,6.81 J5.A7 | J5.B7 33.76,7.06 | 33.76,7.06 33.76,10.83 32.74,11.85 D6.1
V_BATT  (via drill 0.3)
  Top 0.559: U4.1 34.7,44.7 34.51,44.89 34.51,46.29 34.82,46.6 35.4,46.6 | 35.4,46.6 U4.3 | 35.4,46.6 35.36,46.64 C17.1 v35.36,50.01 | MEAS1.2 MEAS1.4
  Horz/GND 0.559: v35.27,87.69 33.08,87.69 32.92,87.86 25.17,87.86 24.93,88.1 23.99,88.1 v23.99,87.97
  Vert 0.559: v35.36,50.01 35.36,87.61 v35.27,87.69 | v23.99,87.97 22.27,89.69 22.27,101.15 20.61,102.81 J10.1
  Bottom 0.305: 20.79,103.06 U7.2 | 20.29,103.06 U7.3 | U10.9 U10.10
  Bottom 0.559: MEAS1.4 17.58,108.23 C15.1 C8.1 17.73,105.19 U10.10 20.36,102.98 J10.1 | D7.A 23.08,101.53 21.81,102.81 J10.1 | J10.1 20.29,103.06 | J10.1 20.79,103.06
VIN  (via drill 0.3)
  Top 0.305: D6.5 v33.24,15.68 | D2.5 45.94,15.56 v46.07,15.68
  Top 0.559: v23.08,73.59 v23.08,98.74 | v63.21,43.11 63.23,43.13 J7.2 | D9.C v47.09,10.06 v47.08,10.05 | MEAS.2 MEAS.4 | D5.AB 53.76,37.1 v54.19,37.53
  Horz/GND 0.559: v39.21,73.47 23.21,73.47 v23.08,73.59 | MEAS.4 41.49,15.05 40.58,15.96 33.42,15.96 33.24,15.78 v33.24,15.68
  Vert 0.559: v39.21,73.47 39.21,73.44 39.18,73.41 39.18,39.33 39.84,38.67 v40.86,38.67 | v63.21,43.11 60.65,40.55 60.65,26.58 51.88,17.82 51.88,14.35 47.77,10.23 47.26,10.23 v47.08,10.05 47.08,10.23 42.38,10.23 41.49,9.34 MEAS.4
  Bottom 0.305: v46.07,15.68 47.08,14.67 v47.08,10.05
  Bottom 0.559: v40.86,38.67 54.19,38.67 | 54.19,38.67 56.26,38.67 57.04,39.46 61.33,39.46 63.21,41.34 v63.21,43.11 | v54.19,37.53 54.19,38.67 | 17.73,98.13 C9.1 17.71,97.84 D7.C v23.08,98.74
  pour Bottom (isolate 0.305, no thermals): 17.75,100.26 17.75,97.72 17.24,97.72 17.24,100.26
ZED-RXI1
  Top 0.178: R9.P5 18.07,31.61 18,31.68 SERIAL1_CONNECTION.5 13.43,31.68 12.66,30.92 5.44,30.92 4.67,31.68 J15.2
ZED-RXI2  (via drill 0.3)
  Top 0.178: J9.3 12.27,6.54 J11.2 12.92,15.17 14.23,16.48 BLUETOOTH_BROADCAST.4 15.78,16.44 v18,16.44 | R4.P3 51.67,28.27 52.26,28.87 52.26,30.56 51.82,31.01 v51.82,31.35
  Horz/GND 0.178: v52.04,35.62 48.68,35.62 47.28,37.02 v20.03,37.02
  Vert 0.178: v20.03,37.02 19.14,37.02 18,35.88 v18,16.44 | v51.82,31.35 51.82,35.41 v52.04,35.62
ZED-TXO1
  Top 0.178: R3.2 21.77,35.11 20.54,35.11 18.38,32.95 13.94,32.95 12.67,31.68 SERIAL1_CONNECTION.2 5.3,31.68 J15.1
ZED-TXO2  (via drill 0.3)
  Top 0.178: R4.P4 51.46,29.07 51.91,29.53 51.91,30.41 49.75,32.57 48.73,32.57 48.23,33.08 48.23,37.37 48.7,37.84 v50.73,37.84 | J9.2 11.02,6.54 J11.3 10.34,7.23 10.34,13.75 10.09,14 BLUETOOTH_BROADCAST.1 11.61,16.48 v11.65,16.44
  Horz/GND 0.178: v9.11,38.03 47.78,38.03 47.97,37.84 v50.73,37.84
  Vert 0.178: v11.65,16.44 10.81,16.44 9.15,18.1 9.15,38 v9.11,38.03
ZED_!SAFE!
  Top 0.178: R2.P6 20.18,24.46 19.27,23.56 J13.2
ZED_FENCE_STAT
  Top 0.178: R4.P1 53.49,26.67 J1.2
ZED_PPS_STAT  (via drill 0.3)
  Top 0.178: R2.P8 21.13,21.35 20.03,20.25 J13.1 | v20.79,38.92 22.32,38.92 25.37,41.97 v28.16,41.97 | R11.2 v43.76,55.18
  Vert 0.178: J13.1 19.33,20.25 20.3,21.23 20.3,36.27 20.79,36.76 v20.79,38.92
  Bottom 0.178: v28.16,41.97 41.37,55.18 v43.76,55.18
ZED_RTK_STAT  (via drill 0.3)
  Top 0.178: R4.P2 51.89,27.47 J1.3 | D3.C v43.84,46.29
  Horz/GND 0.178: v53.56,40.96 53.37,41.14 44.35,41.14 43.84,41.65 v43.84,46.29
  Vert 0.178: J1.3 52.42,30.29 52.42,32.62 53.56,33.76 v53.56,40.96

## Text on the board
Top: v13
Dimension: Route / Out | Route / Out
tPlace: + | -
tDocu: Board thickness is 1.6mm | 4 Layer Board | No clean process | Top PCB surface to inside lid: 11.9mm | Top PCB surface to inside lid: 11.9mm | Inside height: 18.5mm | Thckness of top cover: 2.25mm | 12x12mm switch height: 8.5mm | Rocker height: 16.7mm | LED Height: 0.8mm | Gap to base switch: 3.4mm | Top Cover thickness: 2.25mm | Recommended air gap: 0.5-1.27mm | Pipe length: 12.08-12.85mm | 12.7mm / 0.5" is common | 10.16mm / 0.4" is common | -ND | -ND | 350-3726-ND (Flat $0.25) | 350-3725-ND (Flat $0.25) | 350-3738-ND (Dome $0.25) | NA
